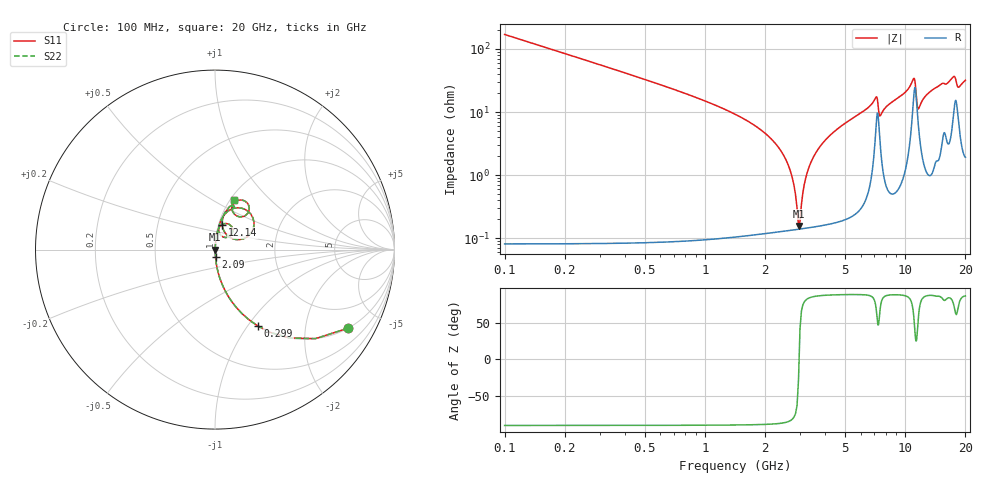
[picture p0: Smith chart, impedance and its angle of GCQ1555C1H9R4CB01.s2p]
!Murata Part Number: GCQ1555C1H9R4CB01
!These Parameters are Measured in Series Mode Connection
!Data Generated on Jan 08, 2026
!  o--ll--o
!Port1  Port2
!  o------o
!Operation Temp=25[degC], DC Bias Voltage=0[V]
!Freq. Start=100[MHz] Stop=20[GHz] 401[Steps]
# Hz S RI R 50
!Freq.(Hz) S11(Real) S11(Imag) S21(Real) S21(Imag) S12(Real) S12(Imag) S22(Real) S22(Imag)
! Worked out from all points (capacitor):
!   401 points, 100 MHz to 20 GHz, reference 50 ohm
!   read as one part in series: C = 9.4 pF near 199.5 MHz
!   lowest |Z| = 156 mohm at 2.936 GHz (marker M1)
!   series resonance near 2.954 GHz, so ESL is about 310 pH
!   S11 on the Smith chart (normalised r, x): 100 MHz: 1.00, -3.38; 299 MHz: 1.00, -1.12; 2.09 GHz: 1.00, -0.08; 12.14 GHz: 1.04, +0.29; 20 GHz: 1.04, +0.64
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1e8  0.7408 -0.4379  0.2592 0.4379  0.2592 0.4379  0.7408 -0.4379
2.99e8  0.2394 -0.426  0.7606 0.426  0.7606 0.426  0.2394 -0.426
7.4675e8  0.0439 -0.2028  0.9561 0.2028  0.9561 0.2028  0.0439 -0.2028
2.09e9  0.00284 -0.0404  0.9972 0.0404  0.9972 0.0404  0.00284 -0.0404
2.5875e9  0.00155 -0.0153  0.9985 0.0153  0.9985 0.0153  0.00155 -0.0153
2.93575e9  0.00139 -0.000719  0.9986 0.000719  0.9986 0.000719  0.00139 -0.000719
3.03525e9  0.00142 0.00313  0.9986 -0.00313  0.9986 -0.00313  0.00142 0.00313
3.23425e9  0.00156 0.0105  0.9984 -0.0105  0.9984 -0.0105  0.00156 0.0105
3.43325e9  0.0018 0.0175  0.9982 -0.0175  0.9982 -0.0175  0.0018 0.0175
4.42825e9  0.00412 0.0487  0.9959 -0.0487  0.9959 -0.0487  0.00412 0.0487
6.7665e9  0.0249 0.1257  0.9751 -0.1257  0.9751 -0.1257  0.0249 0.1257
7.1645e9  0.0783 0.1412  0.9217 -0.1412  0.9217 -0.1412  0.0783 0.1412
7.51275e9  0.0355 0.0765  0.9645 -0.0765  0.9645 -0.0765  0.0355 0.0765
1.005e10  0.0521 0.1942  0.9479 -0.1942  0.9479 -0.1942  0.0521 0.1942
1.099525e10  0.1838 0.2137  0.8162 -0.2137  0.8162 -0.2137  0.1838 0.2137
1.159225e10  0.0746 0.0742  0.9254 -0.0742  0.9254 -0.0742  0.0746 0.0742
1.21395e10  0.0402 0.1384  0.9598 -0.1384  0.9598 -0.1384  0.0402 0.1384
1.338325e10  0.0515 0.1988  0.9485 -0.1988  0.9485 -0.1988  0.0515 0.1988
1.67165e10  0.1128 0.2664  0.8872 -0.2664  0.8872 -0.2664  0.1128 0.2664
1.756225e10  0.1811 0.2576  0.8189 -0.2576  0.8189 -0.2576  0.1811 0.2576
1.8408e10  0.1156 0.1915  0.8844 -0.1915  0.8844 -0.1915  0.1156 0.1915
2e10  0.1058 0.2788  0.8942 -0.2788  0.8942 -0.2788  0.1058 0.2788
